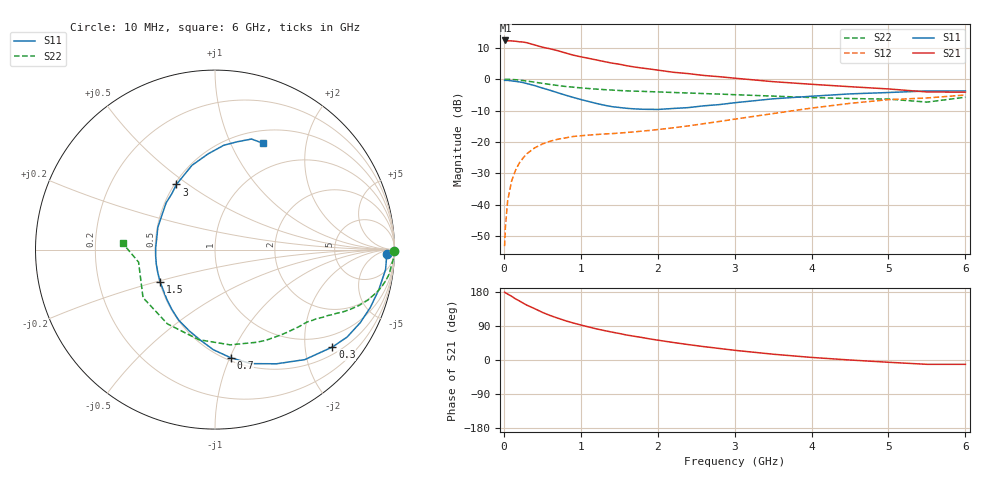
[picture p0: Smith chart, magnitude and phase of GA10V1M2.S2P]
! Infineon Technologies  Discrete & RF Semiconductors
! BF775
! Si NPN RF Bipolar Junction Transistor in SOT23
! VCE = 10 V  IC = 1.2 mA
! Common Emitter S-Parameters:  May  1996
# GHz  S  MA  R  50
!  f  S11  S21  S12  S22
! GHz  MAG  ANG  MAG  ANG  MAG  ANG  MAG  ANG
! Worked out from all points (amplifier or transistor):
!   36 points, 10 MHz to 6 GHz, reference 50 ohm
!   highest |S21| = 12.3 dB at 20 MHz (marker M1)
!   |S21| within 3 dB of that: start of sweep to 658.3 MHz
!   unconditionally stable (mu >= 1): 1.408 GHz to 3.345 GHz
!   at 250 MHz: K = 0.22, MSG = 18.4 dB, |S12| = -25.1 dB
!   at 1.4 GHz: K = 1.00, MSG = 11.2 dB, |S12| = -17.3 dB
!   at 6 GHz: K = 0.96, MSG = 0.5 dB, |S12| = -5.0 dB
!   S11 on the Smith chart (normalised r, x): 10 MHz: 35, -19; 300 MHz: 0.67, -2.62; 700 MHz: 0.53, -1.01; 1.5 GHz: 0.50, -0.21; 3 GHz: 0.51, +0.45; 6 GHz: 0.65, +1.33
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0.01  0.9572 -1.4  4.098 179.0  0.0022 90.0  0.9999 -0.5
0.02  0.9567 -2.9  4.131 177.4  0.0044 89.4  0.9913 -1.0
0.05  0.9569 -6.7  4.082 174.0  0.0117 84.5  0.9961 -2.7
0.1  0.9395 -13.8  4.063 168.3  0.0237 82.7  0.9864 -5.3
0.15  0.9236 -20.4  4.02 161.5  0.0351 77.1  0.98 -8.0
0.25  0.8827 -33.5  3.898 150.2  0.0557 69.8  0.9515 -12.5
0.3  0.8499 -39.7  3.798 144.6  0.0651 66.8  0.9328 -14.7
0.5  0.7226 -61.7  3.229 125.8  0.093 55.7  0.8593 -21.3
0.6  0.6661 -72.5  3.047 117.6  0.1028 51.5  0.8242 -23.8
0.7  0.6085 -81.8  2.84 110.5  0.1105 48.3  0.7938 -25.9
0.9  0.5133 -98.7  2.414 97.8  0.1224 43.7  0.7455 -29.1
1.1  0.4422 -117.2  2.148 87.3  0.1287 41.4  0.7103 -32.0
1.3  0.3866 -133.8  1.912 78.0  0.1342 40.9  0.682 -34.5
1.5  0.3543 -149.7  1.731 70.0  0.1387 41.5  0.6605 -37.1
1.9  0.3308 178.5  1.45 55.6  0.1529 44.3  0.6331 -43.0
2.2  0.3416 158.9  1.289 46.3  0.168 47.0  0.6142 -48.0
3  0.4218 120.6  1.037 25.6  0.231 50.5  0.5664 -65.7
3.5  0.4867 105.3  0.913 15.3  0.2836 48.8  0.5375 -80.9
4.5  0.5833 85.2  0.759 0.0  0.4123 38.3  0.4915 -122.6
5  0.6132 78.4  0.699 -6.0  0.4723 30.2  0.4821 -146.3
5.5  0.6489 71.7  0.626 -11.4  0.5021 20.5  0.4315 -170.7
6  0.6496 65.9  0.621 -11.4  0.5597 15.6  0.5162 176.0
